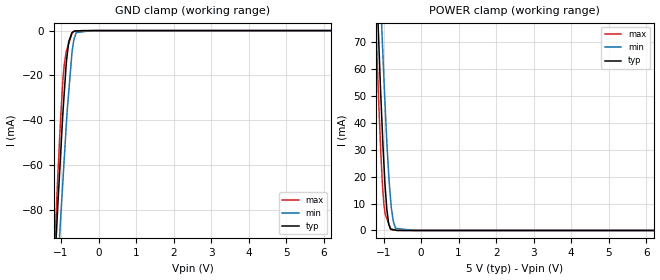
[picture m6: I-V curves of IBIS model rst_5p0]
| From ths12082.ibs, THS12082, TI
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|   rst_5p0 Model
[Model]   rst_5p0
Model_type   Input
Vinl = 0.6
Vinh = 2.6
|   typ   min   max
|   (nom PVT)   (fast PVT)   (slow PVT)
C_comp   9.672e-13   9.597e-13   9.787e-13
| Where nom  PVT is Nominal Process, 5V, 27C
|   Fast PVT is Strong Process,  5.25V, -55C
|   Slow PVT is Weak Process,   4.75V, 125C
[Voltage Range]   5   4.75   5.25
|Ambient Temperature   25   125   -55
|Junction Temperature
[Temperature Range]   27   125   -55
[Power Clamp Reference]   5   4.75   5.25
[GND Clamp Reference]   0   0   0
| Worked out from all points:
|   GND clamp passes 1 mA (typ) near -0.71 V on its own axis
|   POWER clamp passes 1 mA (typ) near -0.83 V on its own axis
[GND Clamp]
|   Voltage   I(typ)   I(min)   I(max)
-5V       -1.643A    -1.563A    -1.767A
-1.306V   -152.4mA   -175mA     -149.2mA
-1.088V   -78.54mA   -106.4mA   -65.44mA
-1.036V   -62.52mA   -90.8mA    -47.5mA
-945mV    -35.33mA   -65.67mA   -20.91mA
-855mV    -13.6mA    -40.69mA   -8.99mA
-795mV    -4.968mA   -27.44mA   -5.848mA
-707.7mV  -971.6uA   -9.742mA   -1.279mA
-640.5mV  -219.1uA   -3.111mA   -156uA
-593.8mV  -169.7uA   -910uA     -144.6uA
-190mV    0A         -23.44nA   -46.27uA
10V       0A         0A         0A
[POWER Clamp]
|   Voltage   I(typ)   I(min)   I(max)
-5V       1.702A     1.703A     1.71A
-1.306V   136.5mA    170mA      116.4mA
-1.129V   70.48mA    104.5mA    47.87mA
-1.059V   45.72mA    79.41mA    25.19mA
-1.029V   35.98mA    69.32mA    16.94mA
-992.2mV  25.31mA    57.06mA    10.05mA
-915mV    8.192mA    33.6mA     4.51mA
-860mV    2.237mA    20.27mA    2.453mA
-798mV    512.4uA    9.233mA    257.7uA
-679.3mV  138.7uA    813.7uA    83.05uA
-190mV    0A         0A         7.728uA
10V       0A         0A         0A
